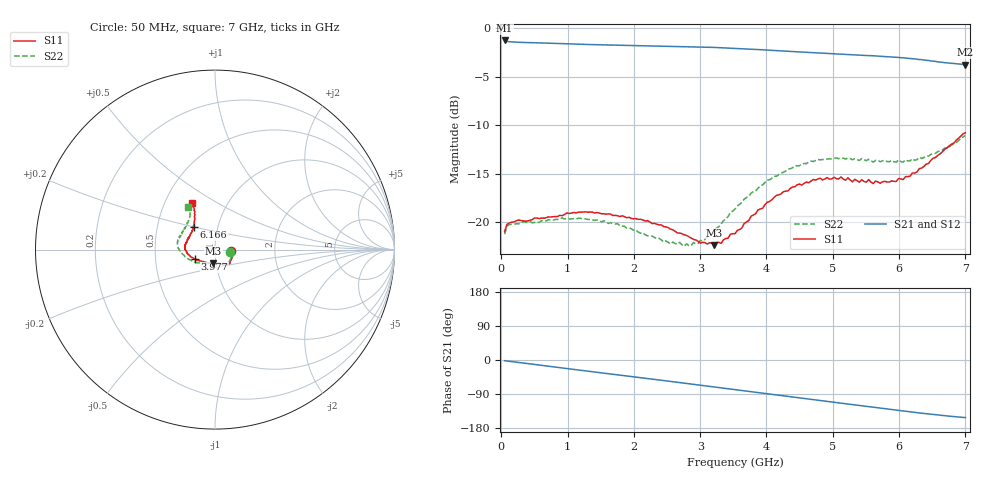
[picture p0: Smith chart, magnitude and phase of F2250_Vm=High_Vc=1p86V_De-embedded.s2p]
! Integrated Device Technology
! Corporate Headquarters
! 6024 Silver Creek Valley Road
! San Jose, CA 95138  USA
! Phone:  1-408-284-8200
! Toll Free:  1-800-223-1366
! Webpage:  http://www.idt.com/
! Timing and RF Division
! 515 Groton Road, Suite 102
! Westford, MA 01886-6024
! Device:  F2250
! Description: Voltage Variable RF Attenuator
! Frequency:  50.0 -  6000.00 MHz
! Package:  3x3 mm Thin QFN Plastic Package: 16 pin
! Ports:  2 RF, 3 DC
!  Pin  1  = GND
!  Pin  2  = NC
!  Pin  3  = RF1  = Port 1
!  Pin  4  = NC
!  Pin  5  = GND
!  Pin  6  = GND
!  Pin  7  = GND
!  Pin  8  = GND
!  Pin  9  = NC
!  Pin 10  = RF2  = Port 2
!  Pin 11  = NC
!  Pin 12  = GND
!  Pin 13  = GND
!  Pin 14  = VCNTRL
!  Pin 15  = VDD
!  Pin 16  = VMODE
! Vcntrl:  1.860 Volts
! Vmode:  +3.300 Volts
! Vdd:  +3.30  Volts
! Current:  1.324 mA
! Data:  The device was measured on a the F2250 evaluation board which has
!  individual transmission lines to the RF pins.  Data was collected
!  using a calibrated network analyzer.  The evaluation board was
!  de-embedded using a TRL calibration technique.
!  The reference plane is the edge of the package pin.
! Misc:  SN 10
!  Action Tracker AT0258
! Date Measured:  2014-11-26
! Date:  2015-10-15  MJV
! Note:
!  Integrated Device Technology supplies this data as a sample of measured
!  data at the package pin for this product.  Your particular data for this
!  product may vary.
!  Data was taken at 25 degrees C.
!  Integrated Device Technology reserves the right to change this data at anytime.
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# GHz S dB R 50
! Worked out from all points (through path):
!   201 points, 50 MHz to 7 GHz, reference 50 ohm
!   highest |S21| = -1.26 dB at 50 MHz (marker M1); lowest = -3.7 dB at 7 GHz (marker M2)
!   group delay of S21, straight-line fit = 61.1 ps
!   lowest |S11| = -22.4 dB at 3.212 GHz (marker M3), VSWR 1.16, Z = 48.5 - j7.37 ohm
!   |S11| at or under -10 dB: start of sweep to end of sweep
!   |S22| runs from -22.5 to -11.1 dB; largest |S21 - S12| = 0.0019
!   S11 on the Smith chart (normalised r, x): 50 MHz: 1.19, -0.02; 3.977 GHz: 0.80, -0.08; 6.166 GHz: 0.77, +0.20; 7 GHz: 0.69, +0.39
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0.05  -21.00 -6.2  -1.26 -1.8  -1.26 -1.8  -21.27 -7.3
0.08475  -20.25 -5.9  -1.35 -2.5  -1.35 -2.5  -20.45 -6.8
0.1195  -20.11 -6.6  -1.39 -3.3  -1.39 -3.3  -20.28 -6.8
0.328  -19.88 -13.7  -1.46 -7.9  -1.47 -7.9  -19.99 -15.3
1.2315  -18.98 -44.5  -1.66 -27.9  -1.66 -27.9  -19.68 -53.0
1.75275  -19.36 -51.4  -1.75 -39.1  -1.75 -39.1  -20.19 -62.9
2.37825  -20.31 -54.0  -1.84 -52.6  -1.84 -52.7  -21.69 -71.7
2.552  -20.74 -57.5  -1.86 -56.5  -1.86 -56.5  -22.29 -78.2
2.86475  -21.67 -68.6  -1.91 -63.5  -1.91 -63.5  -22.44 -95.0
3.07325  -22.14 -83.4  -1.95 -68.2  -1.95 -68.2  -21.81 -110.7
3.21225  -22.37 -97.3  -1.98 -71.3  -1.98 -71.3  -20.86 -121.8
3.525  -21.22 -125.9  -2.07 -78.4  -2.08 -78.5  -18.68 -140.5
3.97675  -18.22 -155.1  -2.24 -88.6  -2.25 -88.7  -15.93 -161.7
4.4285  -16.36 -170.4  -2.42 -98.6  -2.43 -98.6  -14.21 -176.4
4.7065  -15.62 -178.6  -2.52 -104.7  -2.52 -104.7  -13.76 177.2
5.054  -15.54 173.0  -2.65 -112.4  -2.65 -112.4  -13.40 169.5
5.5405  -15.63 157.0  -2.83 -123.1  -2.82 -123.1  -13.54 157.9
5.61  -16.04 156.0  -2.84 -124.5  -2.84 -124.6  -13.82 157.0
5.85325  -15.88 145.8  -2.95 -129.8  -2.95 -129.9  -13.78 149.9
6.166  -15.27 133.5  -3.12 -136.7  -3.12 -136.8  -13.69 141.2
6.54825  -13.35 122.3  -3.42 -144.5  -3.42 -144.7  -12.92 128.9
7  -10.79 116.1  -3.75 -152.0  -3.76 -152.1  -11.09 122.2
